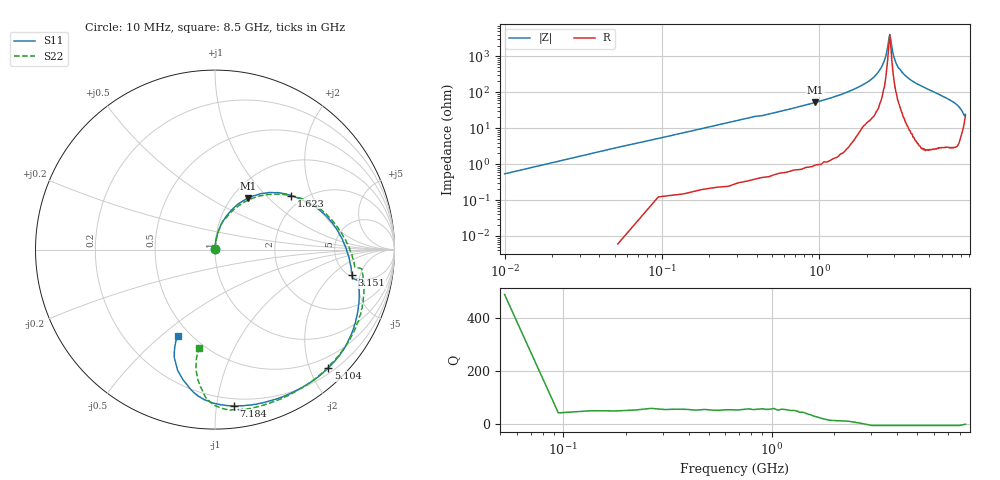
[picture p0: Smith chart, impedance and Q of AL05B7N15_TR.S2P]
!AVX Corporation
!PN: AL05B7N15*TR
!Description: Air Core Inductor, 7.15nH, 7 Turns
!Agilent Technologies,E5071C,MY46102230,A.09.54
!Date: Mon Sep 03 16:21:56 2012
!Data & Calibration Information:
!Freq	S11:SOLT2(ON)	S21:SOLT2(ON)	S12:SOLT2(ON)	S22:SOLT2(ON)
# Hz S dB R 50
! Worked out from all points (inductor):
!   201 points, 10 MHz to 8.5 GHz, reference 50 ohm
!   read as 1/Y11, port 2 shorted: L = 8.71 nH near 52.45 MHz
!   highest Q = 56.5 at 943.9 MHz (marker M1), where L = 8.8 nH
!   self-resonance near 2.769 GHz
!   S11 on the Smith chart (normalised r, x): 10 MHz: 1.00, +0.01; 1.623 GHz: 1.73, +1.42; 3.151 GHz: 5.19, -3.75; 5.104 GHz: 0.29, -2.31; 7.184 GHz: 0.15, -1.12; 8.5 GHz: 0.43, -0.57
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1e7  -47.07 84.6  -0.01 -0.4  0.03 -0.3  -46.73 84.0
5.245e7  -32.60 85.7  -0.01 -2.0  0.02 -2.1  -32.59 86.1
9.49e7  -27.62 84.8  -0.02 -3.6  -0.01 -3.6  -27.59 84.2
1.3735e8  -24.45 83.6  -0.04 -5.1  -0.01 -5.2  -24.37 82.5
2.2225e8  -20.36 80.7  -0.06 -8.2  -0.05 -8.2  -20.39 79.9
3.9205e8  -15.64 74.8  -0.16 -14.4  -0.15 -14.4  -15.61 73.9
9.439e8  -9.37 57.2  -0.61 -32.6  -0.61 -32.7  -9.38 55.5
1.4533e9  -6.34 41.0  -1.30 -49.2  -1.29 -49.3  -6.34 39.6
1.6231e9  -5.68 35.4  -1.58 -54.7  -1.57 -54.7  -5.60 34.8
2.2174e9  -3.84 17.6  -2.66 -71.8  -2.65 -71.9  -3.71 17.4
2.85415e9  -2.59 -2.1  -3.88 -89.5  -3.87 -89.6  -2.53 1.0
3.1513e9  -2.19 -10.6  -4.48 -97.2  -4.47 -97.3  -2.15 -6.1
3.4909e9  -1.47 -18.1  -5.98 -103.9  -5.97 -104.0  -1.42 -12.6
4.255e9  -0.96 -32.4  -7.62 -118.6  -7.62 -118.6  -0.99 -27.3
5.104e9  -0.79 -46.2  -8.73 -134.5  -8.73 -134.5  -0.85 -44.4
5.6983e9  -0.81 -56.0  -9.15 -146.1  -9.15 -146.1  -0.82 -57.2
6.3775e9  -0.92 -67.9  -9.30 -159.0  -9.30 -159.0  -0.84 -70.9
7.09915e9  -1.10 -81.5  -8.77 -172.7  -8.77 -172.7  -0.90 -82.8
7.18405e9  -1.14 -83.2  -8.68 -174.4  -8.67 -174.4  -0.94 -84.0
7.86325e9  -1.89 -98.5  -6.85 166.9  -6.85 166.8  -1.67 -93.6
8.2453e9  -3.25 -108.0  -5.51 150.2  -5.51 150.1  -3.00 -98.1
8.5e9  -5.63 -113.2  -4.42 132.9  -4.43 132.9  -5.09 -99.0
